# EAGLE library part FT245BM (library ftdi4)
USB FIFO 2nd Generation USB FIFO (USB <-> Parallel)
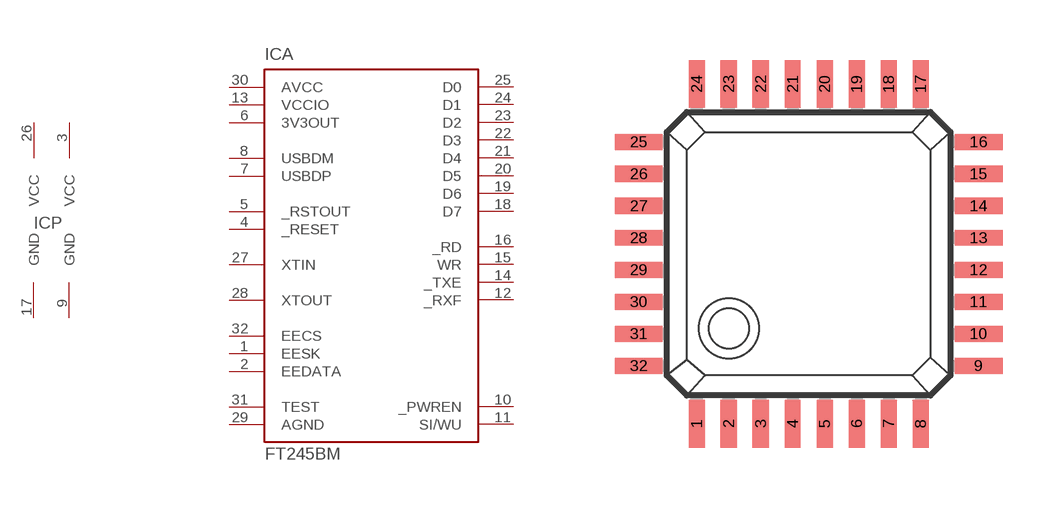
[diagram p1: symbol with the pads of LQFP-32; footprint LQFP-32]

Designator prefix IC; gates A=FT245BM P=2VCC2GND

## FT245BM  [LQFP-32]
1  A:EESK  out
2  A:EEDATA
3  P:VCC  pwr
4  A:_RESET  in
5  A:_RSTOUT  out
6  A:3V3OUT  out
7  A:USBDP
8  A:USBDM
9  P:GND  pwr
10  A:_PWREN  out
11  A:SI/WU  in
12  A:_RXF  out
13  A:VCCIO  pwr
14  A:_TXE  out
15  A:WR  in
16  A:_RD  in
17  P:GND  pwr
18  A:D7
19  A:D6
20  A:D5
21  A:D4
22  A:D3
23  A:D2
24  A:D1
25  A:D0
26  P:VCC  pwr
27  A:XTIN  in
28  A:XTOUT  out
29  A:AGND  pwr
30  A:AVCC  pwr
31  A:TEST  in
32  A:EECS

## Footprint LQFP-32 (pad centres in mm)
Quad Flat Package 32 LD LQFP Source: ds232b12.pdf http://www.ftdichip.com
smd 0.4 x 1.2: 1 -2.8,-4.25; 2 -2,-4.25; 3 -1.2,-4.25; 4 -0.4,-4.25; 5 0.4,-4.25; 6 1.2,-4.25; 7 2,-4.25; 8 2.8,-4.25; 17 2.8,4.25; 18 2,4.25; 19 1.2,4.25; 20 0.4,4.25; 21 -0.4,4.25; 22 -1.2,4.25; 23 -2,4.25; 24 -2.8,4.25
smd 1.2 x 0.4: 9 4.25,-2.8; 10 4.25,-2; 11 4.25,-1.2; 12 4.25,-0.4; 13 4.25,0.4; 14 4.25,1.2; 15 4.25,2; 16 4.25,2.8; 25 -4.25,2.8; 26 -4.25,2; 27 -4.25,1.2; 28 -4.25,0.4; 29 -4.25,-0.4; 30 -4.25,-1.2; 31 -4.25,-2; 32 -4.25,-2.8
